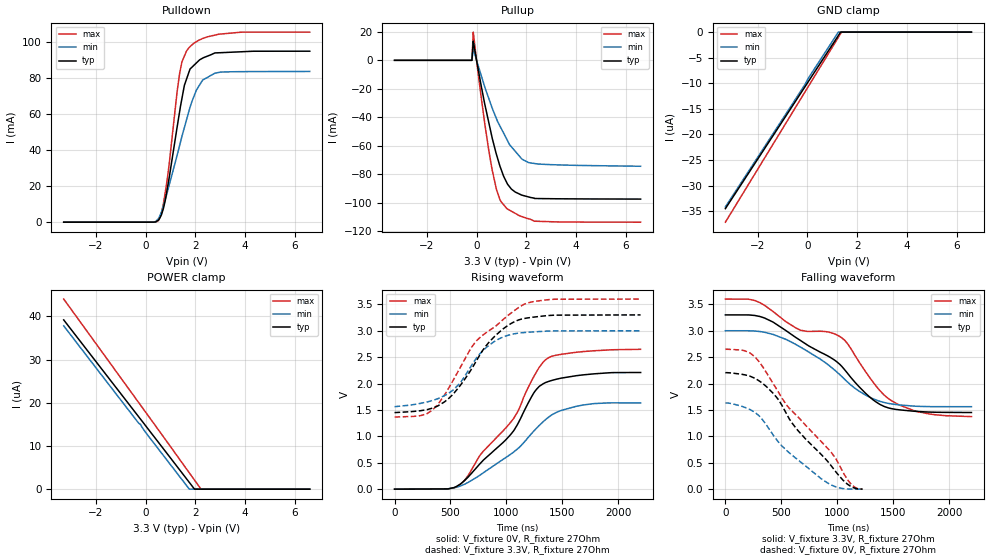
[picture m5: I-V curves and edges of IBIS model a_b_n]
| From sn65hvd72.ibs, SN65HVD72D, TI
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[Model]   a_b_n
Model_type   I/O
Polarity   Non-Inverting
Enable   Active-High
Vinl = 0.8
Vinh = 2.0
Vmeas = 1.65
Vref = 1.65
Cref = 50pF
Rref = 27
|   typ   min   max
|   (nom PVT)   (fast PVT)   (slow PVT)
C_comp   1.239e-11   1.188e-11   1.335e-11
|ON state : BUFFER OUTPUT TURNED HIGH
|C_comp   1.548e-11   1.500e-11   1.704e-11
|OFF state: BUFFER IN HIGH IMPEDANCE
|C_comp   9.313e-12   8.774e-12   9.661e-12
| Where nom  PVT is Nominal Process, 3.3V, 27C
|   Fast PVT is Strong Process,  3.6V, -40C
|   Slow PVT is Weak Process,   3V, 125C
[Voltage Range]   3.3   3   3.6
[Temperature Range]   27   125   -40
[Pullup Reference]   3.3   3   3.6
[Pulldown Reference]   0   0   0
[Power Clamp Reference]   3.3   3   3.6
[GND Clamp Reference]   0   0   0
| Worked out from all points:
|   slope of the pulldown table from 0 to 0.495 V, typ, clamps not added: 498 ohm
|   slope of the pullup table from 0 to 0.495 V, typ, clamps not added: 11.3 ohm
|   falling waveform, V_fixture 3.3V, R_fixture 27Ohm: 20-80 % time 660ns typ, 547ns min, 849ns max; typ from 3.3 V to 1.45 V
|   rising waveform, V_fixture 0V, R_fixture 27Ohm: 20-80 % time 483ns typ, 539ns min, 510ns max; typ from 0 V to 2.21 V
|   rising waveform, V_fixture 3.3V, R_fixture 27Ohm: 20-80 % time 381ns typ, 332ns min, 485ns max; typ from 1.45 V to 3.3 V
|   falling waveform, V_fixture 0V, R_fixture 27Ohm: 20-80 % time 499ns typ, 446ns min, 607ns max; typ from 2.2 V to 0.001 V
[Pulldown]
|   Voltage   I(typ)   I(min)   I(max)
-3.3V     -1.604nA   -10.59nA   0A
478.8mV   854.1uA    1.46mA     485.5uA
633.6mV   4.157mA    5.701mA    5.209mA
828mV     15.47mA    14.57mA    20.22mA
1.278V    54.06mA    37.94mA    74.06mA
1.451V    68.27mA    47.35mA    88.61mA
1.554V    75.96mA    52.52mA    92.24mA
1.782V    85.03mA    63.83mA    97.48mA
1.922V    86.9mA     69.27mA    99.2mA
2.283V    91.04mA    78.8mA     102mA
2.781V    93.97mA    82.73mA    103.9mA
6.6V      94.94mA    83.7mA     105.6mA
[GND Clamp]
|   Voltage   I(typ)   I(min)   I(max)
-3.3V     -34.49uA   -34.15uA   -37.14uA
-579mV    -14.26uA   -13.86uA   -15.52uA
-117mV    -10.82uA   -10.38uA   -11.85uA
93mV      -9.253uA   -8.6uA     -10.18uA
1.245V    -683.2nA   -4.053nA   -1.025uA
1.337V    -1.528nA   0A         -296.1nA
1.372V    0A         0A         -16.67nA
6.6V      0A         0A         0A
[Pullup]
|   Voltage   I(typ)   I(min)   I(max)
-3.3V     0A         0A         0A
-186mV    0A         0A         0A
-133.2mV  13.33mA    8.265mA    19.81mA
61.2mV    -5.892mA   -3.527mA   -8.761mA
338.4mV   -31.41mA   -19.2mA    -45.44mA
633.6mV   -54.91mA   -33.77mA   -77.41mA
795.6mV   -65.81mA   -40.76mA   -90.26mA
939.6mV   -74.23mA   -46.06mA   -97.67mA
1.21V     -85.62mA   -55.2mA    -103.9mA
1.554V    -92.43mA   -63.79mA   -107.4mA
2.091V    -95.87mA   -71.78mA   -111.2mA
6.6V      -97.38mA   -74.35mA   -113.6mA
[POWER Clamp]
|   Voltage   I(typ)   I(min)   I(max)
-3.3V     39.2uA     37.82uA    44.02uA
-309mV    16.95uA    15.47uA    20.25uA
-213mV    16.24uA    15.03uA    19.49uA
18mV      14.52uA    12.98uA    17.65uA
1.752V    1.576uA    18.34nA    3.788uA
1.96V     23.06nA    0A         2.123uA
2.225V    0A         0A         12nA
6.6V      0A         0A         0A
[Ramp]
R_load = 27
|   typ   min   max
dV/dt_r   1.3255/4.82484e-07   0.980086/5.39774e-07   1.58885/5.09675e-07
dV/dt_f   1.10898/6.61233e-07  0.862702/5.46253e-07   1.33541/8.49123e-07
[Falling Waveform]
V_fixture = 3.3V
V_fixture_min = 3V
V_fixture_max = 3.6V
R_fixture = 27Ohm
|   Time   V(typ)   V(min)   V(max)
0s        3.3V       3V         3.6V
264ns     3.289V     2.995V     3.572V
427.9ns   3.162V     2.929V     3.361V
669.5ns   2.818V     2.693V     3.011V
1.024us   2.363V     2.168V     2.89V
1.092us   2.194V     2.028V     2.756V
1.262us   1.799V     1.772V     2.199V
1.424us   1.563V     1.639V     1.773V
1.72us    1.471V     1.569V     1.468V
2.2us     1.452V     1.562V     1.374V
[Rising Waveform]
|Vcc
V_fixture = 0V
V_fixture_min = 0V
V_fixture_max = 0V
R_fixture = 27Ohm
|   Time   V(typ)   V(min)   V(max)
0s        268uV      251.4uV    294.5uV
476.4ns   5.374mV    7.481mV    4.341mV
595.1ns   107.5mV    65.74mV    104mV
660.4ns   234.6mV    130.7mV    264.9mV
768.5ns   492.3mV    273.1mV    654.5mV
1.066us   1.109V     704.8mV    1.344V
1.253us   1.846V     1.117V     2.16V
1.379us   2.041V     1.367V     2.491V
1.689us   2.165V     1.595V     2.606V
2.2us     2.209V     1.634V     2.648V
[Rising Waveform]
V_fixture = 3.3V
V_fixture_min = 3V
V_fixture_max = 3.6V
R_fixture = 27Ohm
|   Time   V(typ)   V(min)   V(max)
0s        1.45V      1.562V     1.366V
233.5ns   1.486V     1.625V     1.393V
342.1ns   1.537V     1.681V     1.505V
532.4ns   1.821V     1.894V     2.093V
725.4ns   2.407V     2.462V     2.792V
815.8ns   2.708V     2.675V     2.958V
911.4ns   2.926V     2.821V     3.1V
1.155us   3.23V      2.965V     3.498V
1.429us   3.295V     2.997V     3.596V
2.2us     3.3V       3V         3.6V
[Falling Waveform]
|Gnd
V_fixture = 0V
V_fixture_min = 0V
V_fixture_max = 0V
R_fixture = 27Ohm
|   Time   V(typ)   V(min)   V(max)
0s        2.204V     1.629V     2.649V
174.2ns   2.165V     1.549V     2.621V
272.7ns   2.088V     1.44V      2.484V
432.4ns   1.804V     1.01V      1.983V
545.4ns   1.432V     737.1mV    1.598V
646.1ns   1.117V     559.4mV    1.376V
851.5ns   669.1mV    206.4mV    913.7mV
986.9ns   330.6mV    43.8mV     579.7mV
1.124us   47.94mV    1.544mV    92.06mV
1.227us   509.5uV    421.7uV    170.1uV
